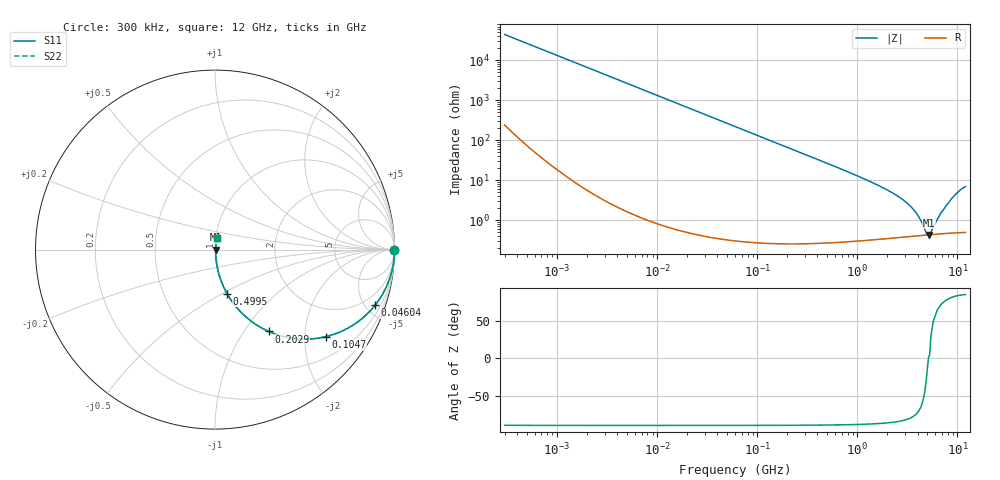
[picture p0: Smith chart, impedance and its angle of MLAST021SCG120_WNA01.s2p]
! MLAST021SCG120_WNA01  S-PARAMETER MODEL  ( General Type )
! Model Generated by TAIYO YUDEN Corporation (http://www.ty-top.com)
! Version 1.0
! TAIYO YUDEN Control No. 220901
! Copyright(c) 2022 TAIYO YUDEN CO.,LTD. All Rights Reserved.
! Product Description (link to TY-COMPAS)
! https://ds.yuden.co.jp/TYCOMPAS/or/detail?pn=MLAST021SCG120JWNA01&u=M
! Products Name : Multilayer Ceramic Capacitors
! Characteristics :
!  Capacitance : 12 pF , Rated Voltage : 25V , TCC : CG / C0G
!  Case Size : 0.25 x 0.125 / 0.0098 x 0.0049 [mm/inch] , Thickness : 0.125 / 0.0049 [mm/inch]
!  (Conditions: Temperature = 25 degC , DC Bias Current/Voltage = 0A / 0V)
! External Node Assignments :
!  1  o---| |---o  2
! GND o---------o GND
! Frequency Range : 0.3MHz  -  12000MHz  [ 401 STEP ]
# MHz S RI R 50
! Freq[MHz].  S11 Real  S11 Imag  S21 Real  S21 Imag  S12 Real  S12 Imag  S22 Real  S22 Imag
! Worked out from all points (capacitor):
!   401 points, 300 kHz to 12 GHz, reference 50 ohm
!   read as one part in series: C = 12 pF near 316.3 kHz
!   lowest |Z| = 425 mohm at 5.141 GHz (marker M1)
!   series resonance near 5.128 GHz, so ESL is about 80 pH
!   S11 on the Smith chart (normalised r, x): 300 kHz: open; 46.04 MHz: 1.01, -5.76; 104.7 MHz: 1.01, -2.53; 202.9 MHz: 1.01, -1.30; 499.5 MHz: 1.01, -0.53; 12 GHz: 1.01, +0.14
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0.3  1 -0.00226  1.73e-05 0.00226  1.73e-05 0.00226  1 -0.00226
1.769972  0.9998 -0.0133  0.00019 0.0133  0.00019 0.0133  0.9998 -0.0133
10.44266  0.9938 -0.0782  0.00621 0.0782  0.00621 0.0782  0.9938 -0.0782
22.51442  0.9719 -0.165  0.0281 0.165  0.0281 0.165  0.9719 -0.165
46.03623  0.8922 -0.3096  0.1078 0.3096  0.1078 0.3096  0.8922 -0.3096
60  0.8297 -0.3752  0.1703 0.3752  0.1703 0.3752  0.8297 -0.3752
104.6549  0.6158 -0.4853  0.3842 0.4853  0.3842 0.4853  0.6158 -0.4853
202.9496  0.2993 -0.456  0.7007 0.456  0.7007 0.456  0.2993 -0.456
353.9943  0.1238 -0.3259  0.8762 0.3259  0.8762 0.3259  0.1238 -0.3259
499.5319  0.0668 -0.2447  0.9332 0.2447  0.9332 0.2447  0.0668 -0.2447
1166.079  0.0144 -0.1059  0.9856 0.1059  0.9856 0.1059  0.0144 -0.1059
2088.533  0.00621 -0.0524  0.9938 0.0524  0.9938 0.0524  0.00621 -0.0524
2870.14  0.00469 -0.0313  0.9953 0.0313  0.9953 0.0313  0.00469 -0.0313
3547.679  0.00426 -0.0192  0.9957 0.0192  0.9957 0.0192  0.00426 -0.0192
4158.869  0.00415 -0.0106  0.9959 0.0106  0.9959 0.0106  0.00415 -0.0106
4875.354  0.00419 -0.00235  0.9958 0.00235  0.9958 0.00235  0.00419 -0.00235
5140.631  0.00423 9.95e-05  0.9958 -9.95e-05  0.9958 -9.95e-05  0.00423 9.95e-05
5420.343  0.00429 0.00234  0.9957 -0.00234  0.9957 -0.00234  0.00429 0.00234
6699.894  0.00464 0.0128  0.9954 -0.0128  0.9954 -0.0128  0.00464 0.0128
8281.503  0.00543 0.0278  0.9946 -0.0278  0.9946 -0.0278  0.00543 0.0278
10236.47  0.00735 0.0505  0.9927 -0.0505  0.9927 -0.0505  0.00735 0.0505
12000  0.00946 0.0674  0.9905 -0.0674  0.9905 -0.0674  0.00946 0.0674
